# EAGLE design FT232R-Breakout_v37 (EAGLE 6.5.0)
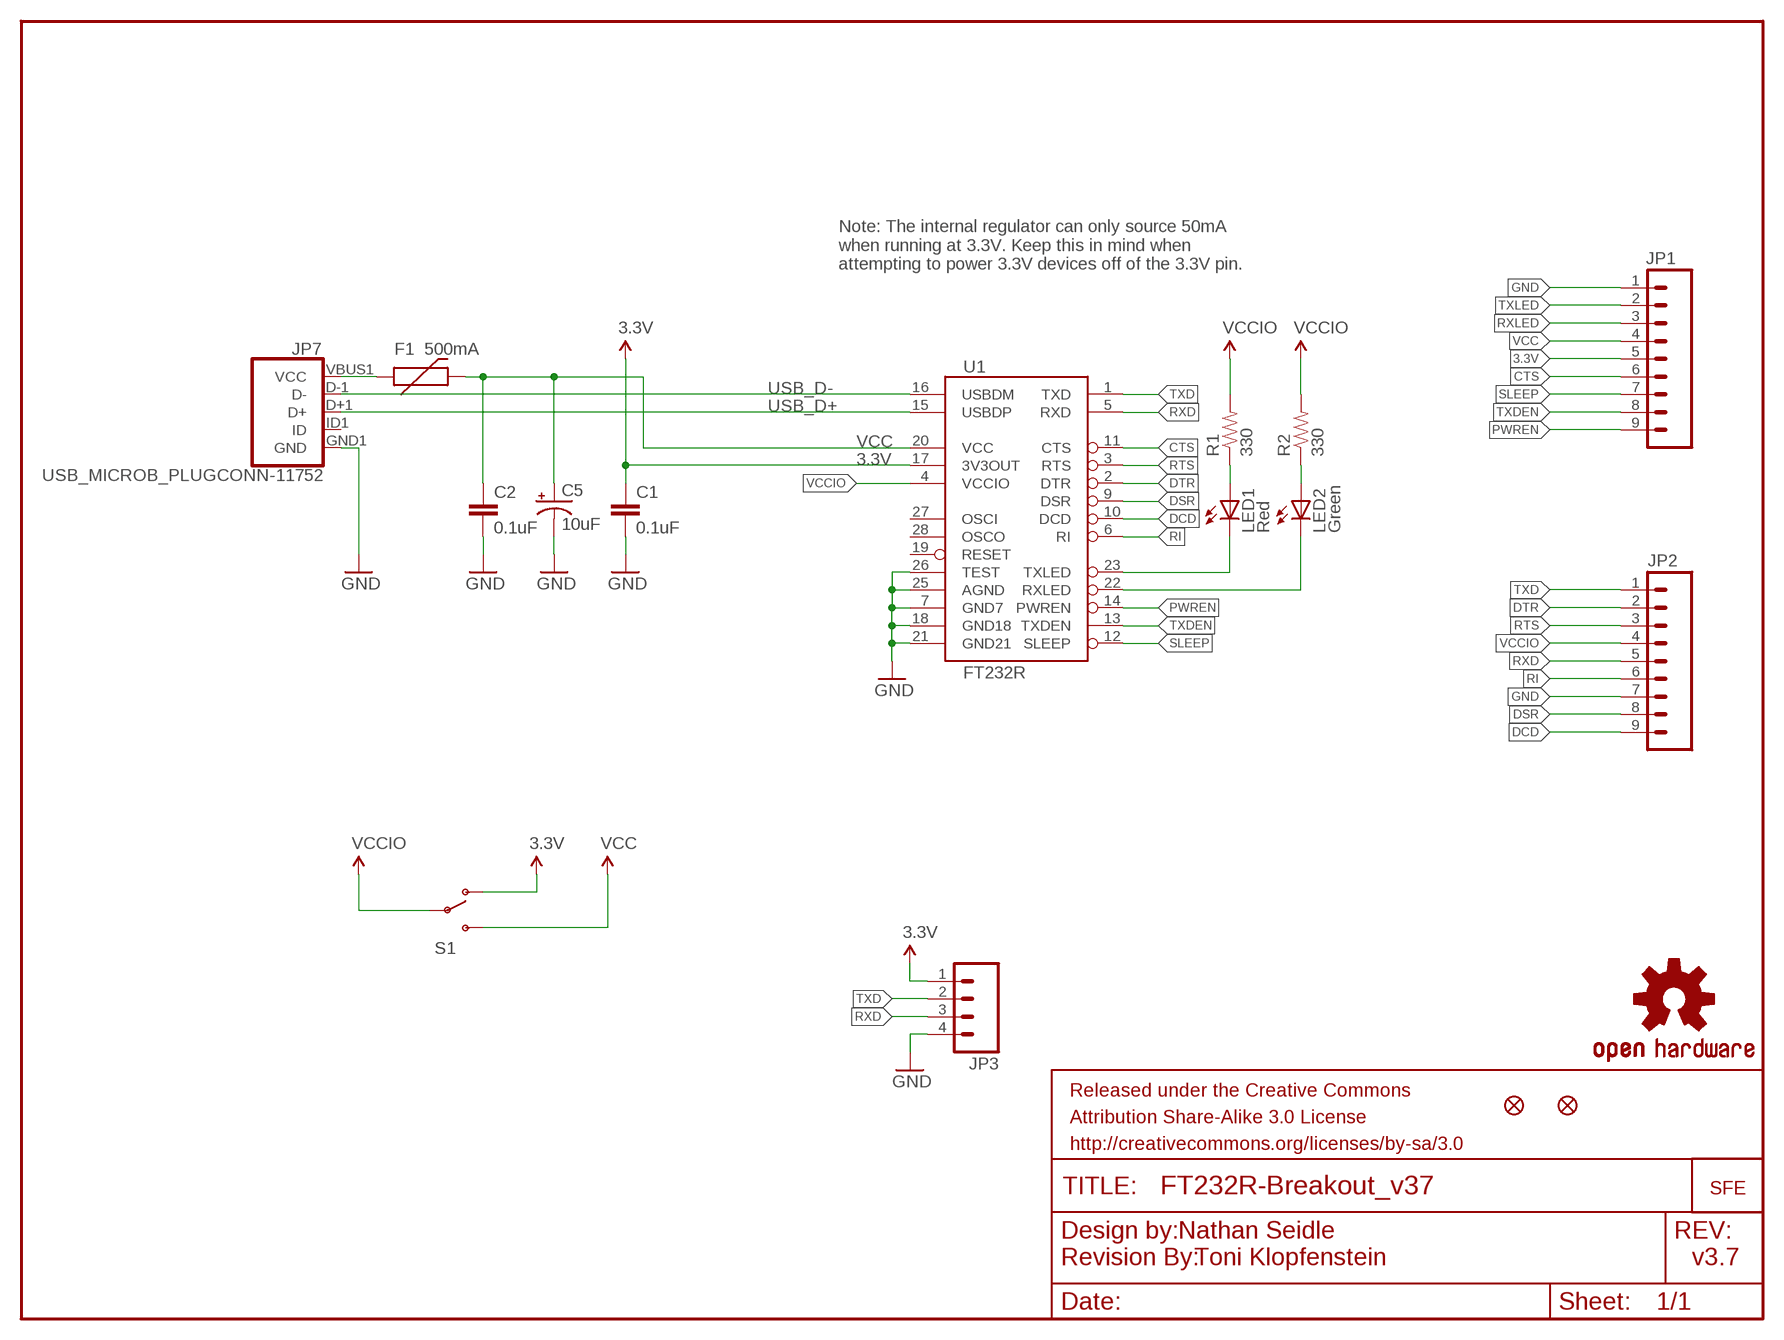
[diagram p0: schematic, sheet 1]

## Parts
C1  0.1uF  0.1UF-25V(+80/-20%)(0603)  [0603-CAP]
C2  0.1uF  0.1UF-25V(+80/-20%)(0603)  [0603-CAP]
C5  10uF  10UF-16V-10%(TANT)  [EIA3216]
F1  500mA  PTCSMD  [PTC-1206]
FRAME1  FRAME-LETTER  [CREATIVE_COMMONS]
JP1  M09  [1X09]
JP2  M09  [1X09]
JP3  M04PTH  [1X04]
JP5  FIDUCIAL1X2  [FIDUCIAL-1X2]
JP6  FIDUCIAL1X2  [FIDUCIAL-1X2]
JP7  USB_MICROB_PLUGCONN-11752  [USB-B-MICRO-SMD_V03]
LED1  Red  LED-RED0603  [LED-0603]
LED2  Green  LED-GREEN0603  [LED-0603]
LOGO1  OSHW-LOGOS  [OSHW-LOGO-S]
R1  330  330OHM1/10W1%(0603)  [0603-RES]
R2  330  330OHM1/10W1%(0603)  [0603-RES]
S1  SWITCH-SPDTSMD  [AYZ0202]
U1  FT232R  FT232RLSSOP  [SSOP28DB]
U$1  REVISION  [REVISION]
U$2  LOGO-SFENEW  [SFE-NEW-WEBLOGO]

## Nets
3.3V [power]: C1.1 JP1.5 JP3.1 S1.1(O) U1.17(3V3OUT)
CTS: JP1.6 U1.11(CTS)
DCD: JP2.9 U1.10(DCD)
DSR: JP2.8 U1.9(DSR)
DTR: JP2.2 U1.2(DTR)
GND [power]: C1.2 C2.2 C5.C(-) JP1.1 JP2.7 JP3.4 JP7.GND1(GND) U1.7(GND7) U1.18(GND18) U1.21(GND21) U1.25(AGND) U1.26(TEST)
N$1: LED1.A R1.1
N$2: LED2.A R2.1
N$3: F1.1 JP7.VBUS1(VCC)
PWREN: JP1.9 U1.14(PWREN)
RI: JP2.6 U1.6(RI)
RTS: JP2.3 U1.3(RTS)
RXD: JP2.5 JP3.3 U1.5(RXD)
RXLED: JP1.3 LED2.C U1.22(RXLED)
SLEEP: JP1.7 U1.12(SLEEP)
TXD: JP2.1 JP3.2 U1.1(TXD)
TXDEN: JP1.8 U1.13(TXDEN)
TXLED: JP1.2 LED1.C U1.23(TXLED)
USB_D+: JP7.D+1(D+) U1.15(USBDP)
USB_D-: JP7.D-1(D-) U1.16(USBDM)
VCC [power]: C2.1 C5.A(+) F1.2 JP1.4 S1.3(S) U1.20(VCC)
VCCIO: JP2.4 R1.2 R2.2 S1.2(P) U1.4(VCCIO)
Unconnected: JP7.ID1(ID) U1.19(RESET) U1.27(OSCI) U1.28(OSCO)

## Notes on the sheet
- Note: The internal regulator can only source 50mA
  when running at 3.3V. Keep this in mind when
  attempting to power 3.3V devices off of the 3.3V pin.
- Nathan Seidle
- Toni Klopfenstein | v3.7

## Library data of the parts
C1 C2 = SparkFun-Capacitors:0.1UF-25V(+80/-20%)(0603): CAP-00810; PROD_ID: CAP-00810
C5 = SparkFun-Capacitors:10UF-16V-10%(TANT): CAP-00811; PROD_ID: CAP-00811
F1 = SparkFun:PTC: Resettable Fuse PTC
FRAME1 = SparkFun-Aesthetics:FRAME-LETTER: Schematic Frame
JP1 JP2 = SparkFun:M09: Header 9 Standard 9-pin 0.1" header. Use with straight break away headers (SKU : PRT-00116), right angle break away headers (PRT-00553), swiss pins (PRT-00743), machine pins (PRT-00117), and female headers (PRT-00115).
JP3 = SparkFun:M04: Header 4 Standard 4-pin 0.1" header. Use with straight break away headers (SKU : PRT-00116), right angle break away headers (PRT-00553), swiss pins (PRT-00743), machine pins (PRT-00117), and female headers (PRT-00115). Molex polarized connector foot print use with SKU : PRT-08231 with associated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
JP5 JP6 = SparkFun:FIDUCIAL: Fiducial Alignment Points
JP7 = SparkFun-Connectors:USB_MICROB_PLUG: USB Micro-B Plug Comes in a variety of packages. Check out Hirose's ZX-x0 line: http://www.hirose.co.jp/cataloge_hp/e24200011.pdf; PROD_ID: CONN-11752
LED1 = SparkFun-LED:LED-RED: Assorted Red LEDs; PROD_ID: DIO-00819; VALUE: RED
LED2 = SparkFun-LED:LED-GREEN: Various green LEDs; PROD_ID: DIO-00821; VALUE: GREEN
LOGO1 = SparkFun-Aesthetics:OSHW-LOGO: Open Source Hardware Logo This logo indicates the piece of hardware it is found on incorporates a OSHW license and/or adheres to the definition of open source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
R1 R2 = SparkFun-Resistors:330OHM1/10W1%(0603): RES-00818; PROD_ID: RES-00818
S1 = SparkFun-Electromechanical:SWITCH-SPDT: SPDT Switch Simple slide switch, Spark Fun Electronics SKU : COM-00102 DPDT SMT slide switch, AYZ0202, SWCH-08179; PROD_ID: SWCH-08179
U1 = SparkFun:FT232RL: USB UART FT232RL 4th Generation USB UART (USB <-> Serial) Controller. Spark Fun Electronics SKU : COM-00650
U$1 = SparkFun-Aesthetics:REVISION
U$2 = SparkFun:LOGO-SFE: Spark Fun Electronics PCB Logo

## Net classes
0 default: width 0.203 mm
1 power: width 0.254 mm

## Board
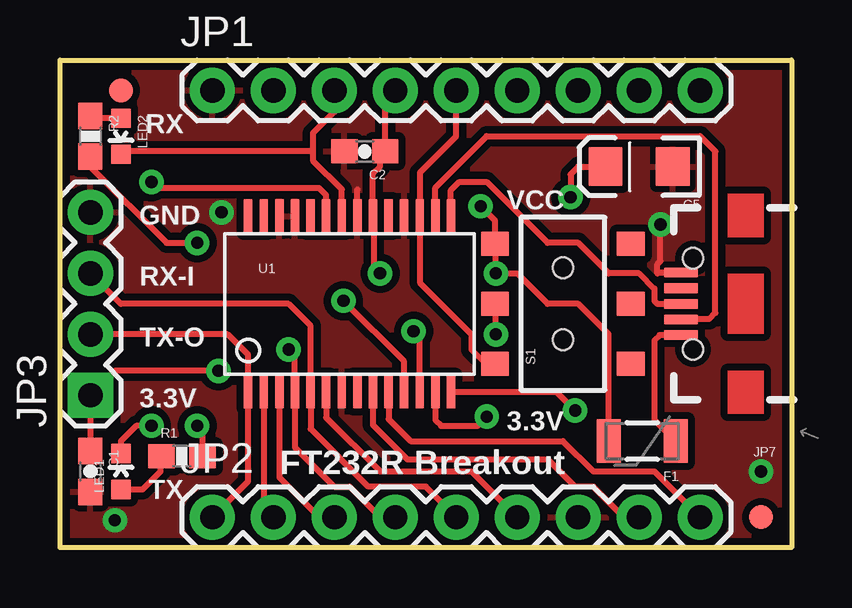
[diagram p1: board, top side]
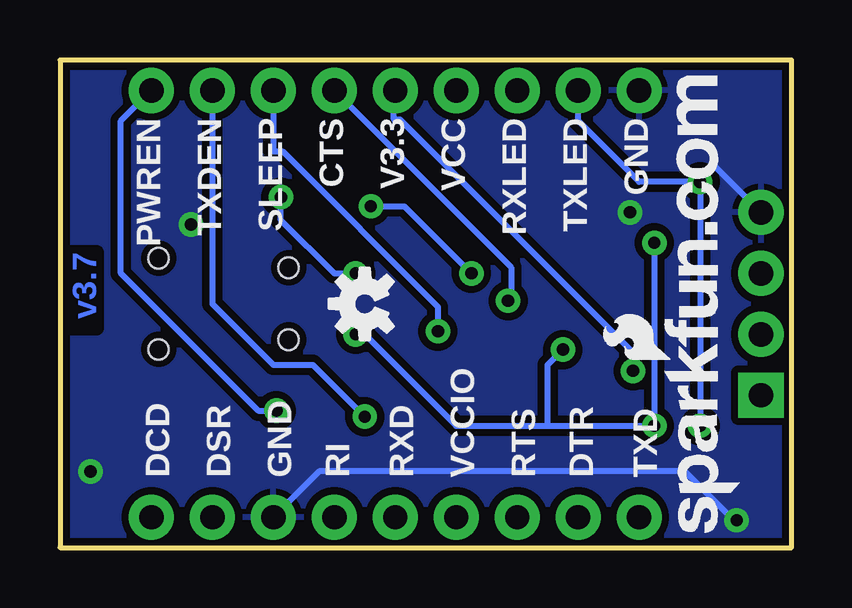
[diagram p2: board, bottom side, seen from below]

Size 30.48 x 20.32 mm. Coordinates in mm from the lower left corner, seen from the top.
Outline: 0,20.32 30.48,20.32 30.48,0 0,0 0,20.32
Copper layers (1*16): Top 0.035mm / dielectric 1.5mm / Bottom 0.035mm
Design rules "SparkFun *": minimum track width 8mil, minimum drill 20mil, track to track 8mil, track to pad 8mil, pad to pad 8mil, via to via 8mil, smd to smd 8mil, copper to edge 10mil, drill to drill 8mil, minimum pad ring 12mil, minimum via ring 10mil, stop-mask expansion 4mil, vias tented up to drill 20mil, thermal gap 10mil

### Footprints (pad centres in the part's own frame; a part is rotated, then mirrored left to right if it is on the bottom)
0603-CAP = smd 1.1 x 1: 1 -0.85,0; 2 0.85,0
EIA3216 = smd 1.4 x 1.6: A 1.4,0; C -1.4,0
PTC-1206 = smd 1 x 1.8: 1 -1.4,0; 2 1.4,0
1X09 = drill 1.016 pad 1.88: 1 0,0; 2 2.54,0; 3 5.08,0; 4 7.62,0; 5 10.16,0; 6 12.7,0; 7 15.24,0; 8 17.78,0; 9 20.32,0
1X04 = drill 1.016 pad 1.88 square: 1 0,0 | drill 1.016 pad 1.88: 2 2.54,0; 3 5.08,0; 4 7.62,0
FIDUCIAL-1X2 = smd 1 x 1: 1 0,0
USB-B-MICRO-SMD_V03 = smd 1.4 x 0.4: D+1 2.7,0; D-1 2.7,0.65; GND1 2.7,-1.3; ID1 2.7,-0.65; VBUS1 2.7,1.3 | hole 0.85: 2.2,1.9; 2.2,-1.9
LED-0603 = smd 0.8 x 0.8: A 0,-0.75; C 0,0.75
0603-RES = smd 1.1 x 1: 1 -0.85,0; 2 0.85,0
AYZ0202 = smd 1 x 1.15: 1 -2.5,2.825; 2 0,2.825; 3 2.5,2.825; 4 -2.5,-2.825; 5 0,-2.825; 6 2.5,-2.825 | hole 0.85: 1.5,0; -1.5,0
SSOP28DB = smd 0.348 x 1.397: 1 -4.225,-3.656; 2 -3.575,-3.656; 3 -2.925,-3.656; 4 -2.275,-3.656; 5 -1.625,-3.656; 6 -0.975,-3.656; 7 -0.325,-3.656; 8 0.325,-3.656; 9 0.975,-3.656; 10 1.625,-3.656; 11 2.275,-3.656; 12 2.925,-3.656; 13 3.575,-3.656; 14 4.225,-3.656; 15 4.225,3.656; 16 3.575,3.656; 17 2.925,3.656; 18 2.275,3.656; 19 1.625,3.656; 20 0.975,3.656; 21 0.325,3.656; 22 -0.325,3.656; 23 -0.975,3.656; 24 -1.625,3.656; 25 -2.275,3.656; 26 -2.925,3.656; 27 -3.575,3.656; 28 -4.225,3.656

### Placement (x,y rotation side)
C1  1.27,3.18 270 top
C2  12.7,16.51 180 top
C5  24.13,15.88 180 top
F1  24.26,4.45 180 top
FRAME1  not placed on the board
JP1  6.35,19.05 0 top
JP2  6.35,1.27 0 top
JP3  1.27,6.35 90 top
JP5  29.21,1.27 0 top
JP6  2.54,19.05 0 top
JP7  28.57,10.16 180 top
LED1  2.54,3.18 0 top
LED2  2.54,17.14 180 top
LOGO1  17.78,10.16 90 bottom
R1  5.08,3.81 0 top
R2  1.27,17.14 270 top
S1  20.96,10.16 90 top
U1  12.07,10.16 0 top
U$1  not placed on the board
U$2  2.16,0.64 90 bottom

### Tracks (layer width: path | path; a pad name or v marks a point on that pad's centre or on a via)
3.3V  (via drill 0.51)
  Top 0.254: 1.4,6.48 JP3.1 | JP1.5 16.51,17.14 14.99,15.62 U1.17 14.99,11.04 17.14,8.89 17.14,8.26 17.78,7.62 18.09,7.62 S1.1 | JP3.1 C1.1 | v6.6,7.37 2.29,7.37 JP3.1
  Bottom 0.254: JP1.5 16.57,18.99 16.57,17.84 16.32,17.84 6.6,8.13 v6.6,7.37
CTS  (via drill 0.51)
  Top 0.254: U1.11 14.34,7.76 v11.81,10.29
  Bottom 0.254: JP1.6 11.68,11.68 11.68,10.41 v11.81,10.29
DCD
  Top 0.254: JP2.9 24.77,3.18 22.23,3.18 20.96,4.45 14.61,4.45 13.69,5.36 U1.10
DSR
  Top 0.254: JP2.8 23.5,1.27 22.23,2.54 21.46,2.54 20.32,3.68 14.48,3.68 13.04,5.12 U1.9
DTR
  Top 0.254: U1.2 8.49,1.67 JP2.2
GND  (via drill 0.51)
  Top 0.254: U1.21 12.39,14.93 | v25.02,13.46 25.02,11.94 24.89,11.81 24.89,11.43 24.92,11.46 JP7.GND1
  Bottom 0.254: JP3.4 1.9,13.97 1.9,14.61 3.18,15.88 | JP2.7 19.68,3.18 4.45,3.18 2.41,1.14 v2.29,1.14
  other vias: 29.21,3.18 6.73,13.97
  pour Bottom (isolate 0.305): 0,0 0,20.32 30.48,20.32 30.48,0
  pour Top (isolate 0.305): 0,0 0,20.32 30.48,20.32 30.48,0
N$1
  Top 0.254: LED1.A 3.44,2.42 4.19,3.18 4.19,3.77 R1.1
N$2
  Top 0.254: 2.64,17.89 LED2.A 1.37,17.89 R2.1
N$3
  Top 0.254: F1.1 24.77,5.34 24.77,8.64 24.99,8.86 JP7.VBUS1
PWREN  (via drill 0.51)
  Top 0.254: U1.14 20.67,6.5 v21.46,5.71
  Bottom 0.254: JP1.9 27.94,17.78 27.94,11.43 22.23,5.71 v21.46,5.71
RI
  Top 0.254: 19.05,1.4 JP2.6 17.14,3.18 13.34,3.18 11.09,5.42 U1.6
RTS
  Top 0.254: U1.3 9.14,2.93 10.79,1.27 JP2.3
RXD
  Top 0.254: JP3.3 2.54,10.16 9.53,10.16 10.44,9.25 U1.5 10.44,4.95 12.85,2.54 15.24,2.54 JP2.5
RXLED
  Top 0.254: U1.22 11.74,14.93 10.54,16.13 10.54,16.51 | 10.54,16.51 2.65,16.51 LED2.C | JP1.3 11.43,18.16 10.54,17.27 10.54,16.51
SLEEP  (via drill 0.51)
  Top 0.254: U1.12 14.99,8.76 v14.73,9.02
  Bottom 0.254: JP1.7 21.59,16.51 21.21,16.51 14.73,10.03 v14.73,9.02
TXD
  Top 0.254: JP2.1 7.84,2.76 U1.1 7.84,8.04 6.99,8.89 JP3.2
TXDEN  (via drill 0.51)
  Top 0.254: U1.13 15.64,5.31 15.88,5.08 17.4,5.08 v17.78,5.46
  Bottom 0.254: JP1.8 24.13,10.16 21.59,7.62 19.94,7.62 v17.78,5.46
TXLED  (via drill 0.51)
  Top 0.254: v3.81,5.08 3.18,5.08 2.54,4.45 LED1.C | U1.23 11.09,14.69 10.79,14.99 4.06,14.99 v3.81,15.24
  Bottom 0.254: v3.81,5.08 v3.81,15.24 6.35,15.24 8.89,17.78 JP1.2
USB_D+
  Top 0.254: U1.15 16.29,14.89 16.64,15.24 17.78,15.24 20.32,12.7 21.59,12.7 22.86,11.43 24.13,11.43 24.77,10.79 24.77,10.29 24.89,10.16 JP7.D+1
USB_D-
  Top 0.254: U1.16 15.64,15 17.78,17.14 26.67,17.14 27.3,16.51 27.3,9.78 27.05,9.53 25.89,9.53 JP7.D-1
VCC  (via drill 0.51)
  Top 0.254: F1.2 22.86,8.89 21.59,10.16 20.32,10.16 19.05,11.43 v18.16,11.43 18.16,12.63 S1.3 18.13,13.62 v17.53,14.22 | JP1.4 13.55,18.63 C2.1 13.34,16.3 13.34,15.88 13.04,15.58 U1.20 13.08,13.78 13.08,11.68 v13.34,11.43 | C5.A 21.59,15.88 21.27,15.56 v21.27,14.61
  Bottom 0.254: v18.16,11.43 19.05,11.43 21.27,13.65 v21.27,14.61 | v13.34,11.43 16.13,14.22 v17.53,14.22
VCCIO  (via drill 0.51)
  Top 0.254: v9.53,8.26 9.79,7.99 U1.4 9.79,4.18 11.43,2.54 12.07,2.54 13.34,1.27 JP2.4 | v5.71,5.08 5.93,5.08 R1.2 | R2.2 1.27,15.88 4.45,12.7 v5.71,12.7 | S1.2 18.13,8.92 v18.16,8.89
  Bottom 0.254: v5.71,12.7 v5.71,5.08 10.16,5.08 | 10.16,5.08 10.16,7.62 v9.53,8.26 | 10.16,5.08 13.97,5.08 17.78,8.89 v18.16,8.89

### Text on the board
Bottom: v3.7
tPlace: RX | GND | VCC | RX-I | TX-O | 3.3V | 3.3V | FT232R Breakout | TX
bPlace: GND | TXLED | RXLED | VCC | V3.3 | CTS | SLEEP | TXDEN | PWREN | TXD | DTR | RTS | VCCIO | RXD | RI | GND | DSR | DCD
tDocu: Nathan Seidle | Toni Klopfenstein

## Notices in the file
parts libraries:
SparkFun-Resistors: Licensing: CC v3.0 Share-Alike You are welcome to use this library for commercial purposes.
SparkFun-Aesthetics: Released under the Creative Commons Attribution Share-Alike 3.0 License
SparkFun-Aesthetics: http://creativecommons.org/licenses/by-sa/3.0
